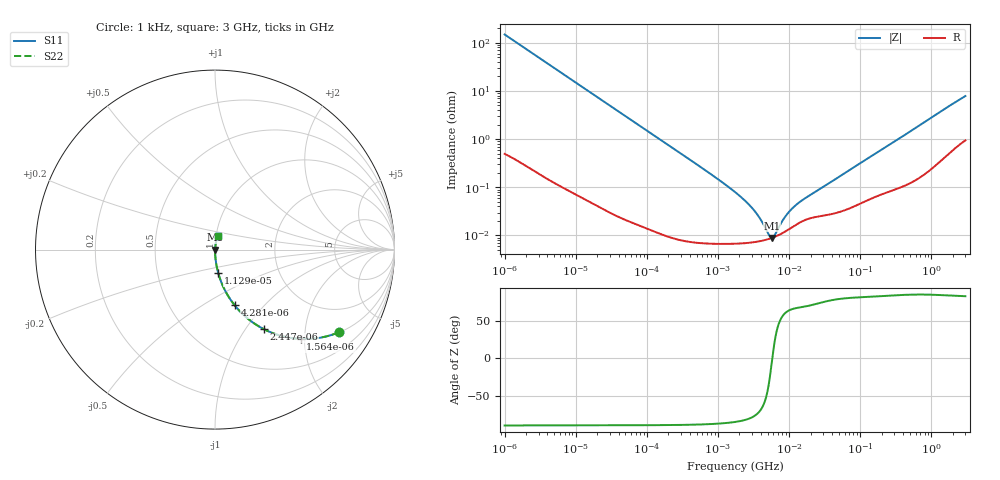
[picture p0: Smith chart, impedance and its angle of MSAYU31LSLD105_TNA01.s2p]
! MSAYU31LSLD105_TNA01  S-PARAMETER MODEL  ( Standard Model )
! Model Generated by TAIYO YUDEN Corporation (http://www.ty-top.com)
! Version 1.0
! TAIYO YUDEN Control No. 220601
! Copyright(c) 2012 TAIYO YUDEN CO.,LTD. All Rights Reserved.
! Product Description (link to TY-COMPAS)
! https://ds.yuden.co.jp/TYCOMPAS/or/detail?pn=MSAYU31LSLD105KTNA01&u=M
! Products Name : Multilayer Ceramic Capacitors
! Characteristics :
!  Capacitance : 1 [uF] , Rated Voltage : 50 [V] , TCC : X5R
!  Case Size : 3.2 x 1.6 / 0.126 x 0.063 [mm/inch] , Thickness : 1.6 / 0.063 [mm/inch]
!  (Conditions: Temperature = 25 [degC] , DC Bias Voltage = 0 [V])
! External Node Assignments :
!  1  o---| |---o  2
! GND o---------o GND
! Frequency Range : 1kHz  -  3GHz  [ 401 STEP ]
# MHZ S RI R 50
! Freq[MHz].  S11 Real  S11 Imag  S21 Real  S21 Imag  S12 Real  S12 Imag  S22 Real  S22 Imag
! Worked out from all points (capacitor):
!   401 points, 1 kHz to 3 GHz, reference 50 ohm
!   read as one part in series: C = 1.07 uF near 1.077 kHz
!   lowest |Z| = 8.93 mohm at 5.711 MHz (marker M1)
!   series resonance near 5.795 MHz, so ESL is about 710 pH
!   S11 on the Smith chart (normalised r, x): 1 kHz: 1.01, -2.98; 1.564 kHz: 1.01, -1.91; 2.447 kHz: 1.00, -1.22; 4.281 kHz: 1.00, -0.70; 11.29 kHz: 1.00, -0.27; 3 GHz: 1.02, +0.16
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0.001  0.6891 -0.4612  0.3109 0.4612  0.3109 0.4612  0.6891 -0.4612
0.001564  0.4766 -0.4976  0.5234 0.4976  0.5234 0.4976  0.4766 -0.4976
0.002447  0.2723 -0.4433  0.7277 0.4433  0.7277 0.4433  0.2723 -0.4433
0.004281  0.1098 -0.3107  0.8902 0.3107  0.8902 0.3107  0.1098 -0.3107
0.006451  0.052 -0.2198  0.948 0.2198  0.948 0.2198  0.052 -0.2198
0.011286  0.018 -0.1304  0.982 0.1304  0.982 0.1304  0.018 -0.1304
0.01216  0.0156 -0.1214  0.9844 0.1214  0.9844 0.1214  0.0156 -0.1214
0.033275  0.00231 -0.0451  0.9977 0.0451  0.9977 0.0451  0.00231 -0.0451
0.147855  0.000215 -0.0102  0.9998 0.0102  0.9998 0.0102  0.000215 -0.0102
0.791611  7.1e-05 -0.00188  0.9999 0.00188  0.9999 0.00188  7.1e-05 -0.00188
1.732051  6.81e-05 -0.000796  0.9999 0.000796  0.9999 0.000796  6.81e-05 -0.000796
3.14518  7.24e-05 -0.000338  0.9999 0.000338  0.9999 0.000338  7.24e-05 -0.000338
3.93371  7.65e-05 -0.000206  0.9999 0.000206  0.9999 0.000206  7.65e-05 -0.000206
5.106836  8.42e-05 -6.53e-05  0.9999 6.53e-05  0.9999 6.53e-05  8.42e-05 -6.53e-05
5.711239  8.9e-05 -7.38e-06  0.9999 7.38e-06  0.9999 7.38e-06  8.9e-05 -7.38e-06
6.387174  9.49e-05 4.99e-05  0.9999 -4.99e-05  0.9999 -4.99e-05  9.49e-05 4.99e-05
8.606987  0.000118 0.000203  0.9999 -0.000203  0.9999 -0.000203  0.000118 0.000203
10.76485  0.000145 0.000319  0.9999 -0.000319  0.9999 -0.000319  0.000145 0.000319
13.97519  0.000184 0.000456  0.9998 -0.000456  0.9998 -0.000456  0.000184 0.000456
21.06097  0.000234 0.000694  0.9998 -0.000694  0.9998 -0.000694  0.000234 0.000694
256.0921  0.000872 0.00754  0.9991 -0.00754  0.9991 -0.00754  0.000872 0.00754
3000  0.0152 0.0761  0.9848 -0.0761  0.9848 -0.0761  0.0152 0.0761
